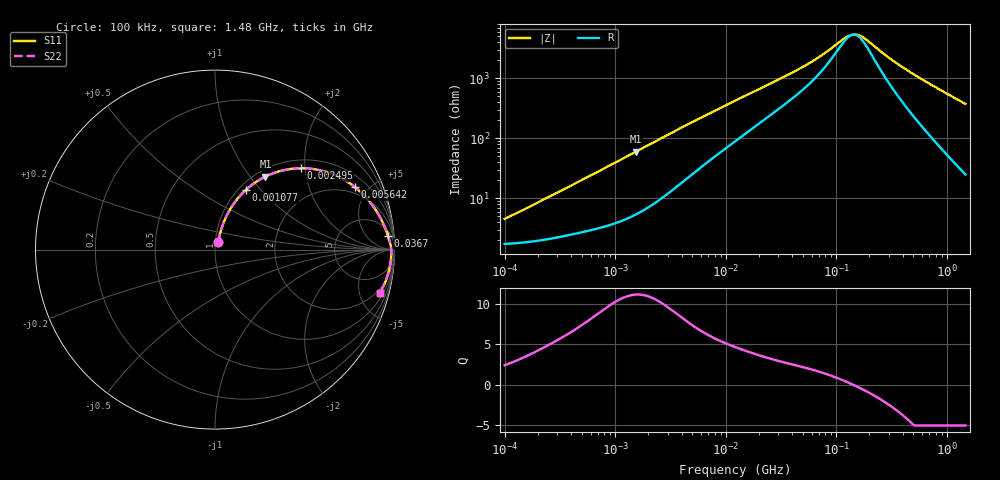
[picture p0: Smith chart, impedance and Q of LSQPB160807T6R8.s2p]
! LSQPB160807T6R8  S-PARAMETER MODEL  ( General Type )
! Model Generated by TAIYO YUDEN Corporation (http://www.ty-top.com)
! Version 1.0
! TAIYO YUDEN Control No. 110308NG25SB-FKC
! Copyright(c) 2011 TAIYO YUDEN CO.,LTD. All Rights Reserved.
! Product Description (link to TY-COMPAS)
! https://ds.yuden.co.jp/TYCOMPAS/or/detail?pn=LSQPB160807T6R8M&u=M
! Products Name : Inductors
! Characteristics :
!  Inductance : 6.8 uH , SRF(min) : 100 MHz , DC Resistance(max) : 2.132 Ohm
!  Rated Current : Saturation :200 mA , Temp Rise : 250 mA (40 degC)
!  Case Size : 1.6 x 0.8 / 0.063 x 0.031 [mm/inch] , Thickness : 0.7 / 0.028 [mm/inch]
!  (Conditions: Temperature = 25 degC , DC Bias Current/Voltage = 0A / 0V)
! External Node Assignments :
!  1  o---GGG---o  2
! GND o---------o GND
! Frequency Range : 0.1MHz  -  1479.677449MHz  [ 402 STEP ]
# MHz S RI R 50
! Freq[MHz].  S11 Real  S11 Imag  S21 Real  S21 Imag  S12 Real  S12 Imag  S22 Real  S22 Imag
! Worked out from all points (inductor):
!   401 points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, 100 kHz to 1.48 GHz, reference 50 ohm
!   read as one part in series: L = 6.6 uH near 130.2 kHz
!   highest Q = 11.1 at 1.543 MHz (marker M1), where L = 6.15 uH
!   self-resonance near 143.3 MHz
!   S11 on the Smith chart (normalised r, x): 100 kHz: 1.03, +0.08; 1.077 MHz: 1.08, +0.84; 2.495 MHz: 1.19, +1.91; 5.642 MHz: 1.60, +4.13; 36.7 MHz: 9, +21; 1.48 GHz: 1.50, -7.46
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0.1  0.0187 0.0403  0.9813 -0.0403  0.9813 -0.0403  0.0187 0.0403
0.237309  0.029 0.0927  0.971 -0.0927  0.971 -0.0927  0.029 0.0927
0.499463  0.0616 0.1819  0.9384 -0.1819  0.9384 -0.1819  0.0616 0.1819
0.751165  0.1047 0.2559  0.8953 -0.2559  0.8953 -0.2559  0.1047 0.2559
1.076754  0.1729 0.3333  0.8271 -0.3333  0.8271 -0.3333  0.1729 0.3333
1.543468  0.2812 0.4068  0.7188 -0.4068  0.7188 -0.4068  0.2812 0.4068
2.494629  0.4802 0.4533  0.5198 -0.4533  0.5198 -0.4533  0.4802 0.4533
3.575915  0.6334 0.4283  0.3666 -0.4283  0.3666 -0.4283  0.6334 0.4283
5.642482  0.7817 0.3466  0.2183 -0.3466  0.2183 -0.3466  0.7817 0.3466
8.088192  0.8563 0.2736  0.1437 -0.2736  0.1437 -0.2736  0.8563 0.2736
12.45974  0.9103 0.1971  0.0897 -0.1971  0.0897 -0.1971  0.9103 0.1971
20.62732  0.9442 0.1292  0.0558 -0.1292  0.0558 -0.1292  0.9442 0.1292
36.69887  0.9639 0.0765  0.0361 -0.0765  0.0361 -0.0765  0.9639 0.0765
60.75563  0.9739 0.044  0.0261 -0.044  0.0261 -0.044  0.9739 0.044
79.11633  0.9774 0.0296  0.0226 -0.0296  0.0226 -0.0296  0.9774 0.0296
118.9866  0.9808 0.0091  0.0192 -0.0091  0.0192 -0.0091  0.9808 0.0091
144.1788  0.9817 -0.000316  0.0183 0.000316  0.0183 0.000316  0.9817 -0.000316
158.7096  0.982 -0.00507  0.018 0.00507  0.018 0.00507  0.982 -0.00507
178.9494  0.9822 -0.0111  0.0178 0.0111  0.0178 0.0111  0.9822 -0.0111
303.4516  0.9814 -0.0412  0.0186 0.0412  0.0186 0.0412  0.9814 -0.0412
608.7327  0.973 -0.1001  0.027 0.1001  0.027 0.1001  0.973 -0.1001
1479.677  0.9193 -0.241  0.0807 0.241  0.0807 0.241  0.9193 -0.241
